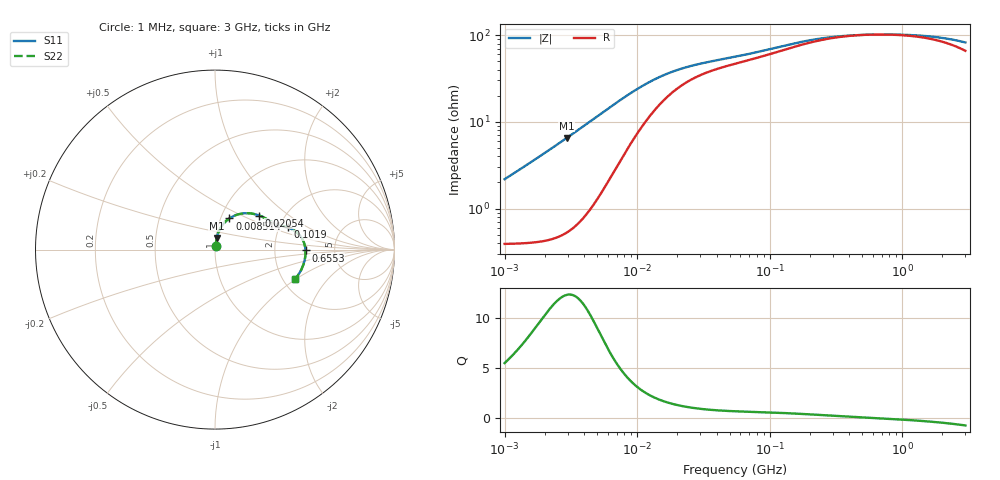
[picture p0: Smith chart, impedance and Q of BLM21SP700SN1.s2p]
! BLM21SP700SN1
# Hz S RI R 50
!Freq.(Hz) S11(Real) S11(Imag) S21(Real) S21(Imag) S12(Real) S12(Imag) S22(Real) S22(Imag)
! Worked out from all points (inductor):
!   401 points, 1 MHz to 3 GHz, reference 50 ohm
!   read as one part in series: L = 342 nH near 1.041 MHz
!   highest Q = 12.3 at 2.947 MHz (marker M1), where L = 351 nH
!   self-resonance near 617.9 MHz
!   S11 on the Smith chart (normalised r, x): 1 MHz: 1.01, +0.04; 8.514 MHz: 1.10, +0.40; 20.54 MHz: 1.50, +0.63; 101.9 MHz: 2.22, +0.67; 655.3 MHz: 3.03, -0.04; 3 GHz: 2.32, -0.98
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1000000  0.00435 0.0213  0.9957 -0.0213  0.9957 -0.0213  0.00435 0.0213
1040844  0.00439 0.0221  0.9956 -0.0221  0.9956 -0.0221  0.00439 0.0221
1462727  0.00496 0.0312  0.995 -0.0312  0.995 -0.0312  0.00496 0.0312
2947212  0.00941 0.0641  0.9906 -0.0641  0.9906 -0.0641  0.00941 0.0641
3823119  0.0145 0.0841  0.9855 -0.0841  0.9855 -0.0841  0.0145 0.0841
5938264  0.0369 0.1306  0.9631 -0.1306  0.9631 -0.1306  0.0369 0.1306
8513927  0.0801 0.1737  0.9199 -0.1737  0.9199 -0.1737  0.0801 0.1737
1.126754e7  0.1315 0.1971  0.8685 -0.1971  0.8685 -0.1971  0.1315 0.1971
1.461624e7  0.185 0.2028  0.815 -0.2028  0.815 -0.2028  0.185 0.2028
2.054061e7  0.2469 0.1899  0.7531 -0.1899  0.7531 -0.1899  0.2469 0.1899
3.065274e7  0.2982 0.1646  0.7018 -0.1646  0.7018 -0.1646  0.2982 0.1646
5.477226e7  0.3485 0.1395  0.6515 -0.1395  0.6515 -0.1395  0.3485 0.1395
1.018679e8  0.404 0.1241  0.596 -0.1241  0.596 -0.1241  0.404 0.1241
1.431579e8  0.4368 0.1094  0.5632 -0.1094  0.5632 -0.1094  0.4368 0.1094
2.094008e8  0.4678 0.0845  0.5322 -0.0845  0.5322 -0.0845  0.4678 0.0845
3.523638e8  0.4937 0.044  0.5063 -0.044  0.5063 -0.044  0.4937 0.044
6.553423e8  0.5043 -0.00463  0.4957 0.00463  0.4957 0.00463  0.5043 -0.00463
8.005644e8  0.5044 -0.0207  0.4956 0.0207  0.4956 0.0207  0.5044 -0.0207
1.171007e9  0.5004 -0.054  0.4996 0.054  0.4996 0.054  0.5004 -0.054
1.645649e9  0.4906 -0.0887  0.5094 0.0887  0.5094 0.0887  0.4906 -0.0887
2.221924e9  0.4741 -0.1244  0.5259 0.1244  0.5259 0.1244  0.4741 -0.1244
3e9  0.4462 -0.1641  0.5538 0.1641  0.5538 0.1641  0.4462 -0.1641
